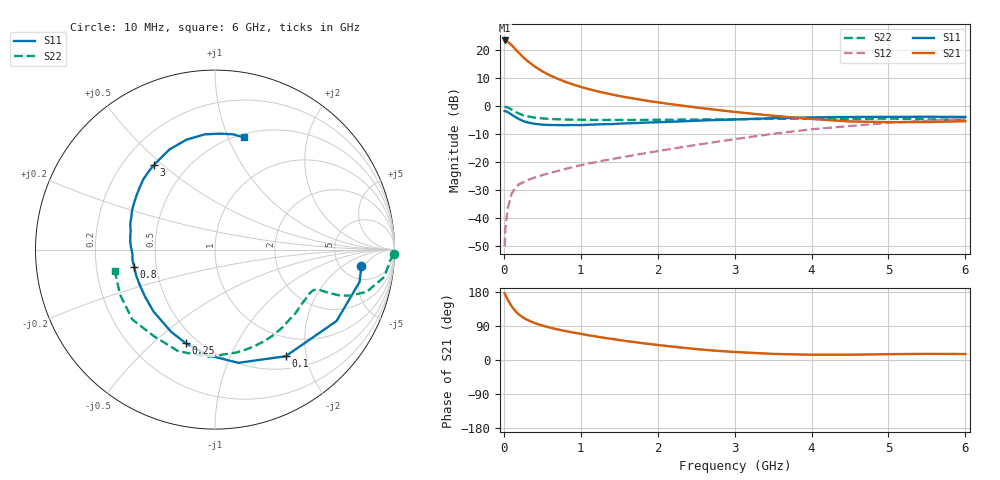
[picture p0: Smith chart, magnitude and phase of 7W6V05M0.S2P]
! Infineon Technologies  Discrete & RF Semiconductors
! BFS17W
! Si NPN RF Bipolar Junction Transistor in SOT323
! VCE = 6 V  IC = 5 mA
! Common Emitter S-Parameters:  August  1999
# GHz  S  MA  R  50
!  f  S11  S21  S12  S22
! GHz  MAG  ANG  MAG  ANG  MAG  ANG  MAG  ANG
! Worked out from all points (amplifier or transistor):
!   36 points, 10 MHz to 6 GHz, reference 50 ohm
!   highest |S21| = 23.5 dB at 10 MHz (marker M1)
!   |S21| within 3 dB of that: start of sweep to 146.1 MHz
!   unconditionally stable (mu >= 1): 577.5 MHz to 2.46 GHz; 5.034 GHz to end of sweep
!   at 250 MHz: K = 0.58, MSG = 22.3 dB, |S12| = -27.1 dB
!   at 1.4 GHz: K = 1.22, MAG = 8.7 dB, |S12| = -18.9 dB
!   at 6 GHz: K = 1.06, MAG = -1.9 dB, |S12| = -4.5 dB
!   S11 on the Smith chart (normalised r, x): 10 MHz: 7.82, -4.25; 100 MHz: 0.68, -1.65; 250 MHz: 0.43, -0.64; 800 MHz: 0.37, -0.09; 3 GHz: 0.33, +0.47; 6 GHz: 0.53, +1.14
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0.01  0.8207 -6.2  14.91 176.1  0.0032 82.4  0.9956 -1.4
0.02  0.8253 -12.6  14.86 171.4  0.0065 88.0  0.976 -3.8
0.05  0.7857 -30.4  14.16 159.1  0.015 76.4  0.9565 -9.1
0.1  0.7126 -56.5  12.33 142.2  0.0272 63.2  0.8781 -15.5
0.15  0.644 -78.4  10.42 128.9  0.0357 56.3  0.7967 -18.8
0.2  0.5883 -94.5  8.836 119.4  0.0409 53.4  0.7383 -20.2
0.25  0.5459 -107.5  7.531 112.1  0.044 50.0  0.6935 -20.7
0.3  0.5189 -118.2  6.536 106.4  0.048 49.9  0.6657 -20.9
0.4  0.4862 -134.7  5.136 97.5  0.0535 50.7  0.6266 -21.1
0.5  0.47 -145.9  4.203 90.9  0.0592 52.1  0.6073 -21.5
0.6  0.4632 -154.8  3.552 85.4  0.0646 54.1  0.5941 -22.3
0.8  0.4608 -167.8  2.728 76.4  0.0764 57.3  0.5803 -25.0
0.9  0.4632 -172.9  2.442 72.5  0.0822 58.6  0.5759 -26.5
1.1  0.4685 178.2  2.03 65.2  0.0952 61.3  0.5725 -30.3
1.3  0.4788 170.4  1.744 58.7  0.108 63.2  0.5692 -34.5
1.6  0.4967 161.3  1.439 49.8  0.1275 65.6  0.569 -41.1
2.2  0.5311 145.4  1.078 35.1  0.1759 69.0  0.5771 -56.3
3  0.5816 125.7  0.793 21.2  0.2591 68.4  0.5857 -78.2
3.5  0.6127 114.6  0.677 16.1  0.3231 65.3  0.5972 -93.1
4.5  0.6446 95.1  0.536 14.0  0.445 53.4  0.5905 -125.2
5.5  0.6504 81.1  0.522 16.2  0.553 40.4  0.5855 -154.7
6  0.6449 75.7  0.542 15.8  0.5953 33.9  0.5701 -167.9
